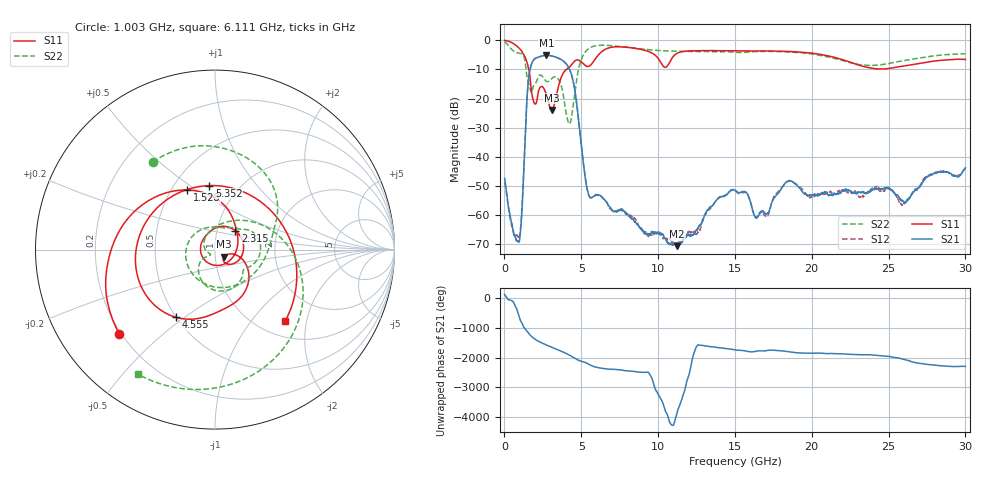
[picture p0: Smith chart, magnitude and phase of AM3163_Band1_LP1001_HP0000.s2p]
!Agilent Technologies,E8364B,MY43040894,A.07.50.67
!Agilent E8364B: A.07.50.67
!Date: Thursday, August 20, 2020 11:28:51
!Correction: S11(Full 2 Port(1,2))
!S21(Full 2 Port(1,2))
!S12(Full 2 Port(1,2))
!S22(Full 2 Port(1,2))
!S2P File: Measurements: S11, S21, S12, S22:
# Hz S  dB  R 50
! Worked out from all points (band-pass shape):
!   3201 points, 10 MHz to 30 GHz, reference 50 ohm
!   highest |S21| = -5.14 dB at 2.728 GHz (marker M1); lowest = -70.6 dB at 11.23 GHz (marker M2)
!   |S21| within 3 dB of the highest: 1.763 GHz to 4.027 GHz (2.264 GHz wide, 78.2 % of centre)
!   lowest |S11| = -23.9 dB at 3.065 GHz (marker M3), VSWR 1.14, Z = 55.1 - j4.44 ohm
!   |S11| at or under -10 dB: 1.585 GHz to 4.026 GHz (2.442 GHz wide, 87 % of centre)
!   |S22| runs from -28.7 to -0.5 dB; largest |S21 - S12| = 0.011
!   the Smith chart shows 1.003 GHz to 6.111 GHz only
!   S11 on the Smith chart (normalised r, x): 1.003 GHz: 0.19, -0.37; 1.528 GHz: 0.60, +0.46; 2.315 GHz: 1.22, +0.27; 4.555 GHz: 0.50, -0.46; 5.352 GHz: 0.73, +0.60; 6.111 GHz: 1.29, -1.50
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1e7  -0.06 -8.8  -47.37 102.5  -48.85 69.1  -0.49 -21.7
5.535688e8  -1.03 -73.7  -64.88 -128.1  -65.15 -138.3  -3.52 -146.5
1.003419e9  -2.97 -138.6  -67.55 -3.6  -66.38 -6.2  -4.45 125.5
1.528244e9  -8.71 115.2  -15.43 -79.3  -15.41 -79.4  -13.70 -93.6
1.931234e9  -21.45 -107.5  -6.54 72.3  -6.54 72.3  -15.37 44.0
2.315481e9  -16.20 43.4  -5.58 -43.8  -5.58 -43.9  -11.90 6.2
2.727844e9  -18.71 -45.0  -5.14 -141.9  -5.15 -142.0  -14.08 -32.8
3.065231e9  -23.86 -38.8  -5.35 145.1  -5.37 145.0  -13.18 -48.4
3.693147e9  -12.77 -35.2  -6.64 11.4  -6.66 11.5  -15.56 -122.0
4.189856e9  -9.37 -84.0  -9.45 -110.6  -9.45 -110.5  -28.50 -132.1
4.555359e9  -7.21 -120.2  -16.36 139.7  -16.32 139.7  -19.33 104.5
5.014581e9  -7.48 165.2  -36.59 33.9  -36.64 34.0  -6.44 -11.4
5.351969e9  -8.92 95.0  -50.29 -27.4  -50.16 -29.4  -3.47 -55.6
6.111091e9  -5.05 -45.7  -53.01 -179.7  -53.25 179.9  -1.76 -121.9
7.676194e9  -2.26 -174.0  -58.46 96.7  -57.88 98.6  -2.26 154.0
1.000979e10  -6.25 69.7  -66.13 19.0  -66.26 -3.9  -3.49 61.7
1.122813e10  -4.49 60.8  -70.61 102.6  -69.96 -85.7  -3.78 18.4
1.5005e10  -3.63 -71.9  -51.54 55.9  -51.26 57.0  -4.14 -93.4
2.000958e10  -4.42 163.5  -53.17 -57.4  -53.84 -59.9  -4.70 136.6
2.275554e10  -7.99 60.4  -52.14 -97.4  -51.74 -100.8  -8.00 21.4
2.500479e10  -9.69 -62.1  -50.80 -162.8  -50.98 -165.6  -7.98 -92.2
3e10  -6.58 105.0  -43.73 -137.3  -43.96 -129.2  -4.63 102.7
